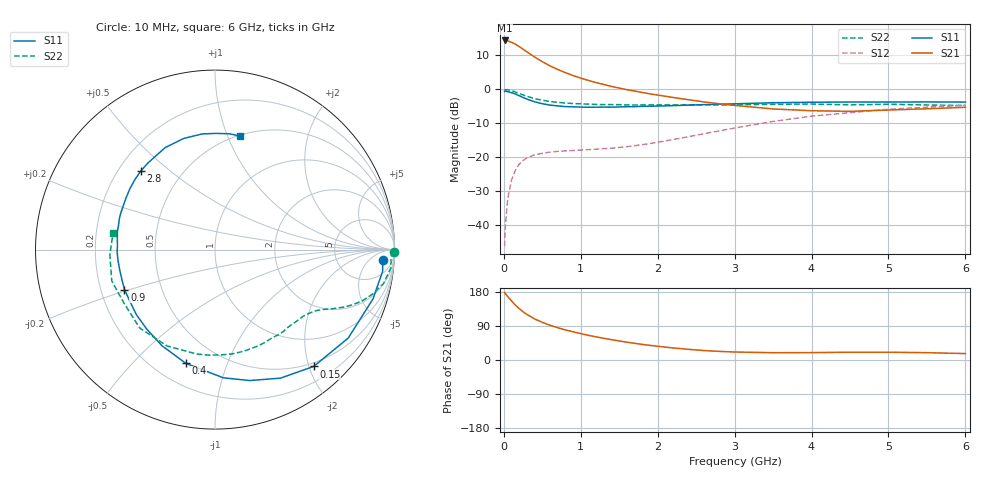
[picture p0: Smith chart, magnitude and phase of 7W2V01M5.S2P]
! Infineon Technologies  Discrete & RF Semiconductors
! BFS17W
! Si NPN RF Bipolar Junction Transistor in SOT323
! VCE = 2 V  IC = 1.5 mA
! Common Emitter S-Parameters:  August  1999
# GHz  S  MA  R  50
!  f  S11  S21  S12  S22
! GHz  MAG  ANG  MAG  ANG  MAG  ANG  MAG  ANG
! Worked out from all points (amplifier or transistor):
!   36 points, 10 MHz to 6 GHz, reference 50 ohm
!   highest |S21| = 14.4 dB at 10 MHz (marker M1)
!   |S21| within 3 dB of that: start of sweep to 275.6 MHz
!   unconditionally stable (mu >= 1): 886.7 MHz to end of sweep
!   at 250 MHz: K = 0.32, MSG = 16.5 dB, |S12| = -21.1 dB
!   at 1.4 GHz: K = 1.34, MAG = 5.7 dB, |S12| = -17.4 dB
!   at 6 GHz: K = 1.11, MAG = -2.3 dB, |S12| = -4.7 dB
!   S11 on the Smith chart (normalised r, x): 10 MHz: 17, -15; 150 MHz: 0.44, -2.08; 400 MHz: 0.33, -0.72; 900 MHz: 0.30, -0.19; 2.8 GHz: 0.29, +0.40; 6 GHz: 0.51, +1.11
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0.01  0.9353 -3.4  5.269 178.2  0.0048 87.6  0.9993 -0.7
0.02  0.942 -7.3  5.267 175.1  0.0097 89.4  0.9818 -2.3
0.05  0.9223 -17.3  5.204 167.4  0.024 81.4  0.9852 -5.9
0.1  0.891 -33.6  4.95 156.0  0.0457 71.6  0.9576 -11.4
0.15  0.8521 -49.8  4.646 144.8  0.0636 62.7  0.9118 -15.8
0.2  0.8038 -63.0  4.281 135.5  0.0781 56.6  0.8674 -19.3
0.25  0.7545 -75.2  3.907 127.3  0.0883 50.6  0.8235 -22.0
0.3  0.7158 -86.3  3.569 120.2  0.0969 46.7  0.7875 -24.0
0.4  0.6538 -104.5  2.997 108.4  0.1076 40.4  0.7279 -27.0
0.5  0.6114 -119.0  2.561 99.3  0.1131 36.4  0.688 -29.0
0.6  0.5837 -130.7  2.216 91.6  0.1178 34.7  0.6606 -30.9
0.7  0.5684 -140.5  1.964 85.2  0.1207 33.6  0.6413 -33.0
0.9  0.5511 -156.2  1.594 74.4  0.1243 33.7  0.6156 -37.2
1.1  0.5427 -168.4  1.351 65.0  0.1283 35.8  0.6032 -42.0
1.4  0.5442 177.6  1.103 53.6  0.1344 40.4  0.5941 -50.1
1.6  0.5531 169.3  0.986 46.9  0.1419 44.3  0.5872 -55.8
2.2  0.5732 149.9  0.757 31.8  0.1809 54.5  0.5885 -74.3
2.8  0.6021 133.1  0.611 22.7  0.2426 58.4  0.5889 -93.8
3.5  0.6326 116.0  0.512 19.2  0.335 55.7  0.5998 -116.5
4.5  0.6484 96.2  0.472 20.5  0.4517 44.1  0.5883 -149.6
5.5  0.6503 82.6  0.515 19.3  0.5441 31.9  0.5865 -177.2
6  0.6473 77.6  0.542 16.9  0.5801 26.2  0.5755 170.7
